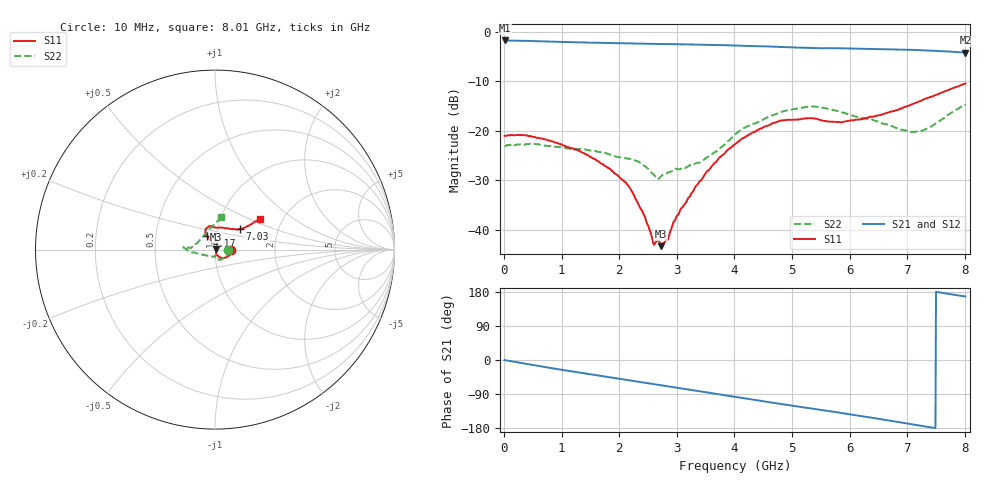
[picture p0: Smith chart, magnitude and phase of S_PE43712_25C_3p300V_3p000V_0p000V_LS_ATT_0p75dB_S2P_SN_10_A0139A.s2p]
! DEVICE ID: PE43712
! File Path: z:\PE43713\PE43713_CHAR_NOM_04292014\AMB\3p300\LS_ATT_0p75dB\PE43713_AMB_3p300V_3p000V_0p000V_LS_ATT_0p75dB_S2P_SN_10_A0139A.s2p
! Serial: 10
! Lot: A0139A
! Temp: 25C
! VDD: 3.300
! VSS: 0.000
! Control_Hi: 3.000
! Control_Lo: 0.000
! Attenuation Step: 0.75dB
! Port 1: RF1
! Port 2: RF2
! ThroughPath:1-2
! IDD: 0.0001466665
! ISS: -1.071e-007
#  Hz  S  RI  R  50
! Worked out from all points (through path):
!   801 points, 10 MHz to 8.01 GHz, reference 50 ohm
!   highest |S21| = -1.74 dB at 10 MHz (marker M1); lowest = -4.2 dB at 8.01 GHz (marker M2)
!   group delay of S21, straight-line fit = 65.8 ps
!   lowest |S11| = -43.3 dB at 2.73 GHz (marker M3), VSWR 1.01, Z = 50.6 + j0.328 ohm
!   |S11| at or under -10 dB: start of sweep to end of sweep
!   |S22| runs from -29.7 to -14.7 dB; largest |S21 - S12| = 0.0027
!   S11 on the Smith chart (normalised r, x): 10 MHz: 1.20, -0.00; 4.17 GHz: 0.91, +0.13; 7.03 GHz: 1.28, +0.31; 8.01 GHz: 1.53, +0.57
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1e7  0.0892 -0.00058  0.8184 -0.00461  0.8181 -0.00429  0.0705 -0.000794
6.9e8  0.0738 -0.0366  0.7616 -0.2494  0.761 -0.2492  0.0616 -0.0358
1.35e9  0.0384 -0.0469  0.6469 -0.4389  0.6464 -0.4387  0.0348 -0.055
1.82e9  0.0188 -0.0374  0.543 -0.5474  0.5427 -0.5471  0.0179 -0.0552
2.14e9  0.00822 -0.0274  0.4625 -0.6095  0.4624 -0.6091  0.00504 -0.0522
2.41e9  0.00641 -0.0136  0.389 -0.6526  0.389 -0.6523  0.00248 -0.0454
2.59e9  0.0067 -0.00306  0.3381 -0.6748  0.3382 -0.6749  -9.58e-05 -0.0367
2.68e9  0.00761 0.00211  0.3135 -0.6854  0.3138 -0.6851  0.00247 -0.0326
2.73e9  0.00604 0.00324  0.3002 -0.6916  0.3001 -0.6916  0.00154 -0.0349
2.83e9  0.00421 0.00674  0.2694 -0.703  0.2698 -0.7029  -0.00353 -0.0374
2.97e9  -0.000228 0.0125  0.2273 -0.7152  0.2275 -0.7151  -0.0108 -0.04
3.36e9  -0.0106 0.0268  0.1069 -0.7341  0.1071 -0.7344  -0.0301 -0.0368
3.74e9  -0.0213 0.0494  -0.00908 -0.7353  -0.00828 -0.7352  -0.0582 -0.0306
4.01e9  -0.0349 0.0645  -0.0919 -0.7224  -0.0913 -0.7222  -0.0891 -0.0229
4.17e9  -0.0439 0.0736  -0.1388 -0.7088  -0.1385 -0.7088  -0.1056 -0.0189
4.78e9  -0.0503 0.1157  -0.3022 -0.6358  -0.3017 -0.6363  -0.1531 -0.00444
5.35e9  -0.0282 0.1311  -0.4259 -0.5397  -0.4256 -0.539  -0.176 0.0124
5.85e9  0.0138 0.1216  -0.5206 -0.4414  -0.5195 -0.4418  -0.1545 0.0105
6.68e9  0.1036 0.1138  -0.6244 -0.2323  -0.6242 -0.2317  -0.1105 0.0265
7.03e9  0.1391 0.1151  -0.6454 -0.1336  -0.6449 -0.1338  -0.0817 0.0551
7.3e9  0.169 0.1237  -0.6476 -0.0557  -0.647 -0.0556  -0.0524 0.0882
8.01e9  0.2485 0.1695  -0.6033 0.1316  -0.6013 0.1303  0.0353 0.1814
